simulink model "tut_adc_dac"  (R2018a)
settings: Solver=VariableStepAuto  StartTime=0.0  StopTime=10.0  RelTol=1e-3
undefined symbols (not defined in the file): adc_data_ch1, adc_data_ch2, adc_data_valid, Bit, Both, bram, c, d, hex2dec, led, Location, Lower, Minimum_Area, out, RED_PITAYA_10, reg, ROACH, ROACH2, rst_cntrl, Unsigned, Upper, Width, xc7z010
libraries: xbsIndex_r4 x149, xps_library x6, casper_library_misc x2
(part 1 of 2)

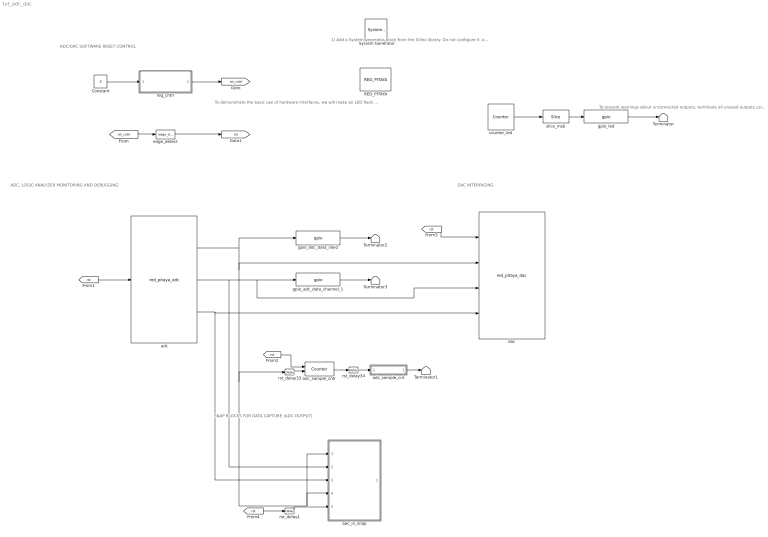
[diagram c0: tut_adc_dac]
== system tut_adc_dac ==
  note: 1) Add a System generator block from the Xilinx library. Do not configure it, add an "XSG core config" to do this for you. 2) Add XSG core config block from the CASPER XPS Blockset. Set it for SKARAB:xc7vx690t with sysclk. sys_clk is an onboard 156.25MHz crystal.
  note: To demonstrate the basic use of hardware interfaces, we will make an LED flash. With the FPGA running at a frequency > 156.25MHz, the most significant bit (msb) of a 27 bit counter will toggle approximately every 1.164 seconds (or quicker). Add a counter (Xilinx Blockset -> Basic Elements -> Counter). Set it for free running, 27 bits, unsigned. Add a slice block to select out the msb (Xilinx Blockset -> Basic Elements -> Slice). Set it for 1 bit wide with offset from top bit at zero. Add a GPIO block (CASPER XPS Blockset -> gpio). Set it to use the Red Pitaya LED bank as output, GPIO bit index 0 (the first LED).
  note: To prevent warnings about unconnected outputs, terminate all unused outputs using a Terminator: Simulink -> Sinks -> Terminator"
  note: ADC/DAC SOFTWARE RESET CONTROL
  note: ADC, LOGIC ANALYZER MONITORING AND DEBUGGING
  note: DAC INTERFACING
  note: SNAP BLOCKS FOR DATA CAPTURE (ADC OUTPUT)
  " System Generator" : xbsIndex_r4/ System Generator  Tag=genX  xilinxfamily=zynq  part=xc7z010  speed=-1  package=clg400  synthesis_tool=XST  clock_wrapper=Clock Enables  directory=/home/hpw1/work/tutorials_devel/vivado_2018/red_pitaya/tut_adc_dac/tut_adc_dac/sysgen  proj_type=Vivado  Synth_file=Vivado Synthesis Defaults  Impl_file=Vivado Implementation Defaults  testbench=off  simulink_period=1  sysclk_period=8  dcm_input_clock_period=10  incr_netlist=off  trim_vbits=Everywhere in SubSystem  dbl_ovrd=According to Block Masks  core_generation=According to Block Masks  run_coregen=off  deprecated_control=off  eval_field=0  block_type=sysgen
  Constant : Constant  Value=0
  RED_PITAYA : xps_library/Platforms/RED_PITAYA  Tag=xps:xsg  hw_sys=RED_PITAYA_10:xc7z010  clk_src=sys_clk  clk_rate=125  sample_period=1  synthesis_tool=XST
  Terminator{,1..3} (4 alike) : Terminator
  adc : xps_library/ADCs/red_pitaya_adc  Tag=xps:red_pitaya_adc  bits=10
  adc_in_snap : Subsystem  Tag=casper:bitsnap  AncestorBlock=casper_library_scopes/bitfield_snapshot  mask(bitsnap){io_names=[adc_data_valid adc_data_ch1 adc_data_ch2], io_widths=[1 10 10], io_bps=0, io_types=[2 1 1], show_format=on, snap_storage=bram, snap_dram_dimm=2, snap_dram_clock=250, snap_nsamples=10, snap_data_width=32, snap_offset=off, snap_circap=off, snap_value=off, snap_ext_arm=off, snap_ext_circ=off, snap_provide_outputs=on, snap_use_dsp48=on, snap_delay=0, extra_names=[c d], extra_widths=[30 2], extra_bps=[0 0], extra_types=[0 0]}
      mask prompts: io_names "Names [msb...lsb]"; io_widths "Bitwidths [msb...lsb]"; io_bps "Binary pts [msb...lsb]"; io_types "Data types [msb...lsb], ufix=0, fix=1, bool=2"; show_format "Print format string?"; snap_storage "Storage medium"; snap_dram_dimm "DRAM dimm"; snap_dram_clock "DRAM clock rate"; snap_nsamples "Number of Samples (2^?)"; snap_data_width "Data width"; snap_offset "Start delay support"; snap_circap "Circular capture support"; snap_value "Extra value capture support"; snap_ext_arm "External arm support"; snap_ext_circ "External circular capture support"; snap_provide_outputs "Provide outputs"; snap_use_dsp48 "Use DSP48s to implement counters"; snap_delay "Pre-snapshot delay"; extra_names "Names [msb...lsb]"; extra_widths "Widths [msb...lsb]"; extra_bps "Binary pts [msb...lsb]"; extra_types "Data types [msb...lsb], ufix=0, fix=1, bool=2"
      mask help: A wrapped snapshot block. Allows specification of inputs to a snapblock word so the toolflow can automatically set up the scope. See documentation for snapshot for explanation of parameters.
      mask init:
      | bitsnap_init(gcb);
  adc_sample_cnt : Subsystem  Tag=xps:sw_reg  AncestorBlock=xps_library/Memory/software_register  mask(swreg){io_dir=To Processor, io_delay=0, init_val=0, sample_period=1, names=reg, bitwidths=32, bin_pts=0, arith_types=0, sim_port=on, show_format=on}
      mask prompts: io_dir "I/O direction"; io_delay "I/O delay"; init_val "Initial Value"; sample_period "Sample period"; names "Bitfield names [msb...lsb]"; bitwidths "Bitfield widths"; bin_pts "Bitfield binary pts"; arith_types "Bitfield types, ufix=0, fix=1, bool=2"; sim_port "Provide sim input/output?"; show_format "Print format string?"
      mask help: A 32-bit software-accessible register. Can be divided into bitfields of varying widths and types using the fields in the block mask.
      mask init:
      | swreg_init(gcb)
  adc_sample_cntr : xbsIndex_r4/Counter  cnt_type=Free Running  cnt_to=1  operation=Up  start_count=0  cnt_by_val=1  arith_type=Unsigned  n_bits=32  bin_pt=0  load_pin=off  rst=on  en=on  explicit_period=on  period=1  use_behavioral_HDL=off  implementation=Fabric  use_rpm=off  dbl_ovrd=off  block_type=counter
  counter_led : xbsIndex_r4/Counter  cnt_type=Free Running  cnt_to=Inf  operation=Up  start_count=0  cnt_by_val=1  arith_type=Unsigned  n_bits=27  bin_pt=0  load_pin=off  rst=off  en=off  explicit_period=on  period=1  use_behavioral_HDL=off  implementation=Fabric  dbl_ovrd=off  block_type=counter
  dac : xps_library/DACs/red_pitaya_dac  Tag=xps:red_pitaya_dac  bits=10
  edge_detect : casper_library_misc/edge_detect  edge=Rising  polarity=Active High  x_in=[0 0.08 0.08 0.16 0.16 0.24 0.24 0.32 0.32 0.4]  y_in="[-1 -1  1  1  1  1  1  1  1  1]"  x_out=[0.6 0.68 0.68 0.76 0.76 0.84 0.84 0.92 0.92 1]  y_out="[-1 -1  1  1 -1 -1 -1 -1 -1 -1]"
  gpio_adc_data_channel_1 : xps_library/IO/gpio  Tag=xps:gpio  io_group_params_forwarded=off  io_group=ROACH:led  io_group_real=gpio  io_group_custom=0  io_dir=out  arith_type="Signed  (2's comp)"  bitwidth=10  bin_pt=0  bit_index=[0 1 2 3 4 5 6 7 8 9]  sample_period=1  use_single_ended=off  use_ddr=off  reg_iob=on  reg_clk_phase=0  termination=None
  gpio_adc_data_valid : xps_library/IO/gpio  Tag=xps:gpio  io_group_params_forwarded=off  io_group=ROACH:led  io_group_real=gpio  io_group_custom=0  io_dir=out  arith_type=Boolean  bitwidth=1  bin_pt=0  bit_index=10  sample_period=1  use_single_ended=off  use_ddr=off  reg_iob=on  reg_clk_phase=0  termination=None
  gpio_led : xps_library/IO/gpio  Tag=xps:gpio  io_group_params_forwarded=on  io_group=ROACH2:led  io_group_real=led  io_group_custom=0  io_dir=out  arith_type=Boolean  bitwidth=1  bin_pt=0  bit_index=0  sample_period=1  use_single_ended=off  use_ddr=off  reg_iob=on  reg_clk_phase=0  termination=None
  reg_cntrl : Subsystem  Tag=xps:sw_reg  AncestorBlock=xps_library/Memory/software_register  mask(swreg){io_dir=From Processor, io_delay=0, init_val=0, sample_period=1, names=rst_cntrl, bitwidths=[1], bin_pts=0, arith_types=[2], sim_port=on, show_format=on}
      mask prompts: io_dir "I/O direction"; io_delay "I/O delay"; init_val "Initial Value"; sample_period "Sample period"; names "Bitfield names [msb...lsb]"; bitwidths "Bitfield widths"; bin_pts "Bitfield binary pts"; arith_types "Bitfield types, ufix=0, fix=1, bool=2"; sim_port "Provide sim input/output?"; show_format "Print format string?"
      mask help: A 32-bit software-accessible register. Can be divided into bitfields of varying widths and types using the fields in the block mask.
      mask init:
      | swreg_init(gcb)
  rst_delay1 : xbsIndex_r4/Delay  rst=off  infoeditControl=Selection of Reset will increase slice count due to use of real FFs and instead of SRLs  en=off  latency=1  reg_retiming=on  dbl_ovrd=off  block_type=delay
  rst_delay33 : xbsIndex_r4/Delay  rst=off  infoeditControl=Selection of Reset will increase slice count due to use of real FFs and instead of SRLs  en=off  latency=2  reg_retiming=on  dbl_ovrd=off  block_type=delay
  rst_delay34 : xbsIndex_r4/Delay  rst=off  infoeditControl=Selection of Reset will increase slice count due to use of real FFs and instead of SRLs  en=off  latency=2  reg_retiming=on  dbl_ovrd=off  block_type=delay
  slice_msb : xbsIndex_r4/Slice  nbits=1  boolean_output=off  mode=Upper Bit Location + Width  bit1=0  base1=MSB of Input  bit0=0  base0=LSB of Input  dbl_ovrd=off  block_type=slice
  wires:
  gpio_led/1 -> Terminator/1
  counter_led/1 -> slice_msb/1
  slice_msb/1 -> gpio_led/1
  Constant/1 -> reg_cntrl/1(sim_1)
  reg_cntrl/1(in_rst_cntrl) -> [rst_cntrl]
  [rst_cntrl] -> edge_detect/1
  edge_detect/1 -> [rst]
  [rst] -> adc/1
  rst_delay34/1 -> adc_sample_cnt/1(out_reg)
  rst_delay33/1 -> adc_sample_cntr/2
  adc_sample_cnt/1(sim_out) -> Terminator1/1
  adc_sample_cntr/1 -> rst_delay34/1
  [rst] -> adc_sample_cntr/1
  adc/1 -> gpio_adc_data_valid/1, adc_in_snap/1(in_adc_data_valid), adc_in_snap/4(we), rst_delay33/1, dac/2
  gpio_adc_data_valid/1 -> Terminator2/1
  gpio_adc_data_channel_1/1 -> Terminator3/1
  [rst] -> dac/1
  rst_delay1/1 -> adc_in_snap/5(trig)
  [rst] -> rst_delay1/1
  adc/2 -> adc_in_snap/2(in_adc_data_ch1), dac/3, gpio_adc_data_channel_1/1
  adc/3 -> adc_in_snap/3(in_adc_data_ch2), dac/4

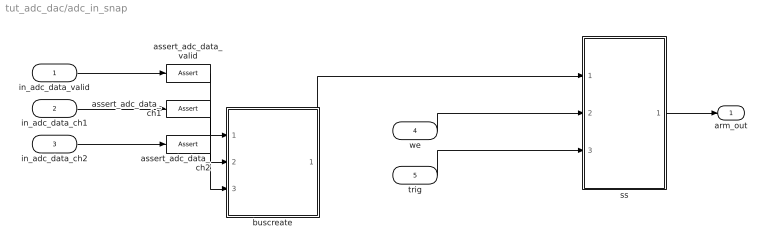
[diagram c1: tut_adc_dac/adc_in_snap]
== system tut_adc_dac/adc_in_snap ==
  in_adc_data_valid : Inport
  in_adc_data_ch1 : Inport  Port=2
  in_adc_data_ch2 : Inport  Port=3
  we : Inport  Port=4
  trig : Inport  Port=5
  assert_adc_data_ch1 : xbsIndex_r4/Assert  assert_type=on  type_source=Explicitly  gui_display_data_type=Fixed-point  arith_type="Signed  (2's comp)"  n_bits=10  bin_pt=0  preci_type=Single  exp_width=8  frac_width=24  assert_rate=off  rate_source=Explicitly  period=1  output_port=on  block_type=assert
  assert_adc_data_ch2 : xbsIndex_r4/Assert  assert_type=on  type_source=Explicitly  gui_display_data_type=Fixed-point  arith_type="Signed  (2's comp)"  n_bits=10  bin_pt=0  preci_type=Single  exp_width=8  frac_width=24  assert_rate=off  rate_source=Explicitly  period=1  output_port=on  block_type=assert
  assert_adc_data_valid : xbsIndex_r4/Assert  assert_type=on  type_source=Explicitly  gui_display_data_type=Boolean  arith_type=Boolean  n_bits=1  bin_pt=0  preci_type=Single  exp_width=8  frac_width=24  assert_rate=off  rate_source=Explicitly  period=1  output_port=on  block_type=assert
  buscreate : Subsystem  AncestorBlock=casper_library_flow_control/bus_create  mask(bus_create){inputNum=3}
      mask prompts: inputNum "Number of inputs:"
      mask init:
      | bus_create_init(gcb,...
      |     'inputNum', inputNum);
  ss : Subsystem  Tag=casper:snapshot  AncestorBlock=casper_library_scopes/snapshot  mask(snapshot){storage=bram, dram_dimm=2, dram_clock=250, nsamples=10, data_width=32, offset=off, circap=off, value=off, ext_arm=off, ext_circ=off, provide_outputs=off, use_dsp48=on}
      mask prompts: storage "Storage medium"; dram_dimm "DRAM dimm"; dram_clock "DRAM clock rate"; nsamples "Number of Samples (2^?)"; data_width "Data width"; offset "Start delay support"; circap "Circular capture support"; value "Extra value capture support"; ext_arm "External arm support"; ext_circ "External circular capture support"; provide_outputs "Provide outputs"; use_dsp48 "Use DSP48s to implement counters"
      mask help: Standard snap block, but with the following optional extras; 1) Optionally delay the fabric trigger by a user-specified number of valids. 2) Capture continuously after a trigger until a stop pulse is received. Data is captured into BRAM continuously, with old data being overwritten until a stop command is received. Then stop capturing when memory is filled. This enables you to get some data before and some data after the stop pulse. Use the 'tr_en_cnt' register to determine where you are in your vector. 'Addr' register's MSb now indicates 'busy capturing'. 3) Optionally capture a value on an i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
      mask init:
      | snapshot_init(gcb, ...
      |     'storage', storage, ...
      |     'dram_dimm', dram_dimm, ...
      |     'dram_clock', dram_clock, ...
      |     'nsamples', nsamples, ...
      |     'data_width', data_width, ...
      |     'offset', offset, ...
      |     'circap', circap, ...
      |     'value', value, ...
      |     'ext_arm', ext_arm, ...
      |     'ext_circ', ext_circ, ...
      |     'provide_outputs', 'off', ...
      |     'use_dsp48', use_dsp48);
  arm_out : Outport
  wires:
  ss/1(arm_out) -> arm_out/1
  buscreate/1(bus_out) -> ss/1(din)
  in_adc_data_valid/1 -> assert_adc_data_valid/1
  assert_adc_data_valid/1 -> buscreate/1(in1)
  in_adc_data_ch1/1 -> assert_adc_data_ch1/1
  assert_adc_data_ch1/1 -> buscreate/2(in2)
  in_adc_data_ch2/1 -> assert_adc_data_ch2/1
  assert_adc_data_ch2/1 -> buscreate/3(in3)
  we/1 -> ss/2(we)
  trig/1 -> ss/3(trig)

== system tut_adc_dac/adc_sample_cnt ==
  out_reg : Inport
  assert_reg : xbsIndex_r4/Assert  assert_type=on  type_source=Explicitly  gui_display_data_type=Fixed-point  arith_type=Unsigned  n_bits=32  bin_pt=0  preci_type=Single  exp_width=8  frac_width=24  assert_rate=off  rate_source=Explicitly  period=1  output_port=on  block_type=assert
  cast_gw : xbsIndex_r4/Convert  gui_display_data_type=Fixed-point  arith_type=Unsigned  n_bits=32  bin_pt=0  float_type=Single  exp_bits=8  fraction_bits=24  quantization=Truncate  overflow=Wrap  en=off  latency=1  pipeline=off  dbl_ovrd=off  block_type=convert
  io_delay : xbsIndex_r4/Delay  rst=off  infoeditControl=Selection of Reset will increase slice count due to use of real FFs and instead of SRLs  en=off  latency=0  reg_retiming=on  dbl_ovrd=off  block_type=delay
  reint1 : xbsIndex_r4/Reinterpret  force_arith_type=on  arith_type=Unsigned  force_bin_pt=on  bin_pt=0  block_type=reinterpret
  tut_adc_dac_adc_sample_cnt_user_data_in : xbsIndex_r4/Gateway Out  inherit_from_input=off  hdl_port=on  rows=1  columns=1  UseAsDAC=off  DACChannel='1'  interface=None  automatic_assignment=on  address_offset=hex2dec('00')  intf_name=''  intf_description=''  timing_constraint=None  locs_specified=off  LOCs={}  io_standard={}  block_type=gatewayout
  sim_out : Outport
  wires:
  io_delay/1 -> cast_gw/1
  cast_gw/1 -> tut_adc_dac_adc_sample_cnt_user_data_in/1
  tut_adc_dac_adc_sample_cnt_user_data_in/1 -> sim_out/1
  out_reg/1 -> assert_reg/1
  assert_reg/1 -> reint1/1
  reint1/1 -> io_delay/1

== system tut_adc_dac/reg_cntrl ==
  sim_1 : Inport
  convert1_1 : DataTypeConversion  OutDataTypeStr=fixdt('ufix1_En0')
  convert2_1 : DataTypeConversion  OutDataTypeStr=fixdt('ufix1_En0')  ConvertRealWorld=Stored Integer (SI)
  gain_1 : Gain
  io_delay : xbsIndex_r4/Delay  rst=off  infoeditControl=Selection of Reset will increase slice count due to use of real FFs and instead of SRLs  en=off  latency=0  reg_retiming=on  dbl_ovrd=off  block_type=delay
  slice_rst_cntrl : xbsIndex_r4/Slice  nbits=1  boolean_output=on  mode=Lower Bit Location + Width  bit1=0  base1=MSB of Input  bit0=0  base0=LSB of Input  dbl_ovrd=off  block_type=slice
  tut_adc_dac_reg_cntrl_user_data_out : xbsIndex_r4/Gateway In  gui_display_data_type=Fixed-point  arith_type=Unsigned  n_bits=32  bin_pt=0  preci_type=Single  exp_width=8  frac_width=24  rows=1  columns=1  quantization="Round  (unbiased: +/- Inf)"  overflow=Saturate  period=1  UseAsADC=off  ADCChannel='1'  interface=None  automatic_assignment=on  address_offset=hex2dec('00')  intf_name=''  intf_description=''  default_value=0  timing_constraint=None  locs_specified=off  LOCs={}  io_standard={}  inherit_from_input=off  hdl_port=on  dbl_ovrd=off  block_type=gatewayin
  in_rst_cntrl : Outport
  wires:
  tut_adc_dac_reg_cntrl_user_data_out/1 -> io_delay/1
  sim_1/1 -> convert1_1/1
  convert1_1/1 -> convert2_1/1
  convert2_1/1 -> gain_1/1
  gain_1/1 -> tut_adc_dac_reg_cntrl_user_data_out/1
  io_delay/1 -> slice_rst_cntrl/1
  slice_rst_cntrl/1 -> in_rst_cntrl/1

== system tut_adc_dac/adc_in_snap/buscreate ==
  in1 : Inport
  in2 : Inport  Port=2
  in3 : Inport  Port=3
  concatenate : xbsIndex_r4/Concat  num_inputs=3  dbl_ovrd=off  block_type=concat
  reinterpret1 : xbsIndex_r4/Reinterpret  force_arith_type=on  arith_type=Unsigned  force_bin_pt=on  bin_pt=0  block_type=reinterpret
  reinterpret2 : xbsIndex_r4/Reinterpret  force_arith_type=on  arith_type=Unsigned  force_bin_pt=on  bin_pt=0  block_type=reinterpret
  reinterpret3 : xbsIndex_r4/Reinterpret  force_arith_type=on  arith_type=Unsigned  force_bin_pt=on  bin_pt=0  block_type=reinterpret
  bus_out : Outport
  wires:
  concatenate/1 -> bus_out/1
  in1/1 -> reinterpret1/1
  reinterpret1/1 -> concatenate/1
  in2/1 -> reinterpret2/1
  reinterpret2/1 -> concatenate/2
  in3/1 -> reinterpret3/1
  reinterpret3/1 -> concatenate/3

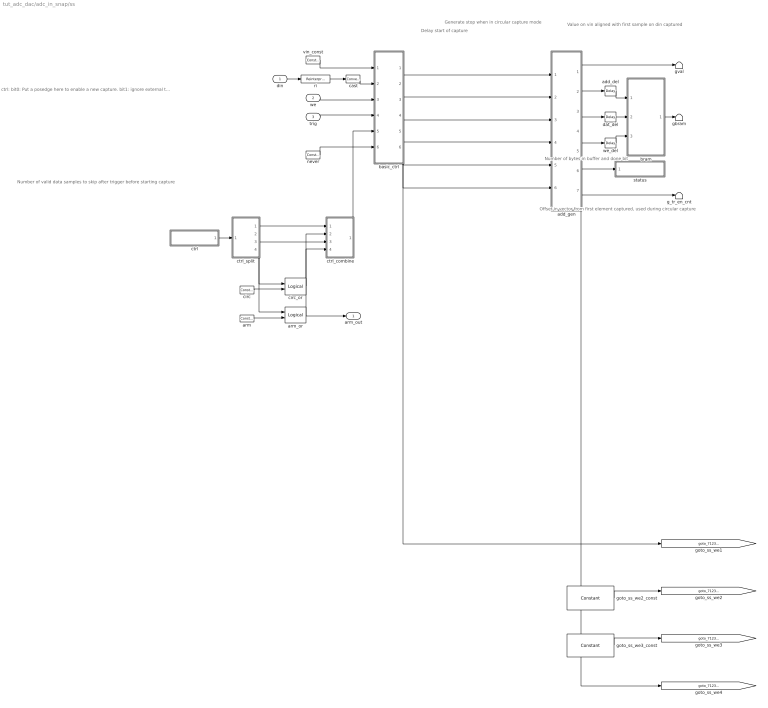
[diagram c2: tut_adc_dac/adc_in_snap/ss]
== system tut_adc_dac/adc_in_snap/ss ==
  note: Generate stop when in circular capture mode
  note: Delay start of capture
  note: ctrl: bit0: Put a posedge here to enable a new capture. bit1: ignore external trigger and trigger immediately. bit2: ignore external write enable and capture on every FPGA clock. bit3: continuously capture data until we get an external stop command.
  note: Offset in vector from first element captured, used during circular capture
  note: Number of bytes in buffer and done bit
  note: Number of valid data samples to skip after trigger before starting capture
  note: Value on vin aligned with first sample on din captured
  din : Inport
  we : Inport  Port=2
  trig : Inport  Port=3
  add_del : xbsIndex_r4/Delay  rst=off  infoeditControl=Selection of Reset will increase slice count due to use of real FFs and instead of SRLs  en=off  latency=1  reg_retiming=on  dbl_ovrd=off  block_type=delay
  add_gen : Subsystem  AncestorBlock=casper_library_scopes/snapshot/add_gen  mask{counter_size=10+2+1, increment=4, nsamples=10, burst_size=0, use_dsp48=on}
      mask prompts: counter_size "Address counter size (2^?)"; increment "Address counter increment"; nsamples "Number of samples (2^?)"; burst_size "Burst size (2^?)"; use_dsp48 "dsp48 counter/s"
      mask init:
      | set_param(gcb,'LinkStatus','inactive');
      | if strcmp(use_dsp48,'on'),
      |     set_param([gcb,'/add_gen'],'implementation','DSP48');
      | else
      |     set_param([gcb,'/add_gen'],'implementation','Fabric');
      | end
  arm : xbsIndex_r4/Constant  const=0  gui_display_data_type=Fixed-point  arith_type=Boolean  n_bits=16  bin_pt=14  preci_type=Single  exp_width=8  frac_width=24  explicit_period=on  period=1  equ=P=C  opselect=C  inp2=PCIN>>17  opr=+  inp1=P  carry=CIN  dbl_ovrd=off  block_type=constant
  arm_or : xbsIndex_r4/Logical  logical_function=OR  inputs=2  en=off  latency=0  precision=Full  arith_type=Unsigned  n_bits=16  bin_pt=0  align_bp=on  dbl_ovrd=off  block_type=logical
  basic_ctrl : Subsystem  AncestorBlock=casper_library_scopes/snapshot/basic_ctrl  mask{dram=off, data_width=32}
      mask prompts: data_width "data width"
      mask init:
      | set_param(gcb,'LinkStatus','inactive');
      | set_param([gcb,'/dram_munge'], 'dram', dram);
  bram : Subsystem  Tag=xps:bram  AncestorBlock=xps_library/Memory/shared_bram  mask{arith_type=Unsigned, addr_width=10, data_width=32, reg_prim_output=off, reg_core_output=off, optimization=Minimum_Area, data_bin_pt=0, init_vals=[0:2^10-1], sample_rate=1}
      mask prompts: arith_type "Output Data Type"; addr_width "Address width"; data_width "Data Width"; reg_prim_output "Register Primitive Output"; reg_core_output "Register Core Output"; data_bin_pt "Data Binary Point"; init_vals "Initial values (simulation only)"; sample_rate "Sample rate"
      mask init:
      | shared_bram_mask;
  cast : xbsIndex_r4/Convert  gui_display_data_type=Fixed-point  arith_type=Unsigned  n_bits=32  bin_pt=0  float_type=Single  exp_bits=8  fraction_bits=24  quantization=Truncate  overflow=Wrap  en=off  latency=0  pipeline=off  dbl_ovrd=off  block_type=convert
  circ : xbsIndex_r4/Constant  const=0  gui_display_data_type=Fixed-point  arith_type=Boolean  n_bits=16  bin_pt=14  preci_type=Single  exp_width=8  frac_width=24  explicit_period=on  period=1  equ=P=C  opselect=C  inp2=PCIN>>17  opr=+  inp1=P  carry=CIN  dbl_ovrd=off  block_type=constant
  circ_or : xbsIndex_r4/Logical  logical_function=OR  inputs=2  en=off  latency=0  precision=Full  arith_type=Unsigned  n_bits=16  bin_pt=0  align_bp=on  dbl_ovrd=off  block_type=logical
  ctrl : Subsystem  Tag=xps:sw_reg  AncestorBlock=xps_library/Memory/software_register  mask(swreg){io_dir=From Processor, io_delay=0, init_val=0, sample_period=1, names=reg, bitwidths=32, bin_pts=0, arith_types=0, sim_port=off, show_format=on}
      mask prompts: io_dir "I/O direction"; io_delay "I/O delay"; init_val "Initial Value"; sample_period "Sample period"; names "Bitfield names [msb...lsb]"; bitwidths "Bitfield widths"; bin_pts "Bitfield binary pts"; arith_types "Bitfield types, ufix=0, fix=1, bool=2"; sim_port "Provide sim input/output?"; show_format "Print format string?"
      mask help: A 32-bit software-accessible register. Can be divided into bitfields of varying widths and types using the fields in the block mask.
      mask init:
      | swreg_init(gcb)
  ctrl_combine : Subsystem  AncestorBlock=casper_library_flow_control/bus_create  mask(bus_create){inputNum=4}
      mask prompts: inputNum "Number of inputs:"
      mask init:
      | bus_create_init(gcb,...
      |     'inputNum', inputNum);
  ctrl_split : Subsystem  AncestorBlock=casper_library_flow_control/bus_expand  mask(bus_expand){mode=divisions of arbitrary size, outputNum=1, outputWidth=[28 1 2 1], outputBinaryPt=0, outputArithmeticType=[0 2 0 2], show_format=on, outputToWorkspace=off, variablePrefix=out, outputToModelAsWell=on}
      mask prompts: outputNum "Number of outputs:"; outputWidth "Output width [msb ... lsb]:"; outputBinaryPt "Output binary point position [msb ... lsb]:"; outputArithmeticType "Output arithmetic type (ufix=0, fix=1, bool=2) [msb ... lsb]:"; show_format "Print format string?"; outputToWorkspace "Output to workspace?"; variablePrefix "Variable name prefix:"; outputToModelAsWell "Output to model as well?"
      mask help: Expands a 'bus' made using a bus_create or Xilinx concat block. The input will be divided into the specified number of outputs with the specified arithmetic types. Divisions are made from most significant bit.
      mask init:
      | bus_expand_init(gcb,...
      |     'mode', mode, ...
      |     'outputNum', outputNum, ...
      |     'outputWidth', outputWidth, ...
      |     'outputBinaryPt', outputBinaryPt, ...
      |     'outputArithmeticType', outputArithmeticType, ...
      |     'show_format', show_format, ...
      |     'outputToWorkspace', outputToWorkspace, ...
      |     'variablePrefix', variablePrefix, ...
      |     'outputToModelAsWell', outputToModelAsWell);
  dat_del : xbsIndex_r4/Delay  rst=off  infoeditControl=Selection of Reset will increase slice count due to use of real FFs and instead of SRLs  en=off  latency=1  reg_retiming=on  dbl_ovrd=off  block_type=delay
  g_tr_en_cnt : Terminator
  gbram : Terminator
  goto_ss_we2_const : xbsIndex_r4/Constant  const=0  gui_display_data_type=Fixed-point  arith_type=Boolean  n_bits=16  bin_pt=14  preci_type=Single  exp_width=8  frac_width=24  explicit_period=on  period=1  equ=P=C  opselect=C  inp2=PCIN>>17  opr=+  inp1=P  carry=CIN  dbl_ovrd=off  block_type=constant
  goto_ss_we3_const : xbsIndex_r4/Constant  const=0  gui_display_data_type=Fixed-point  arith_type=Boolean  n_bits=16  bin_pt=14  preci_type=Single  exp_width=8  frac_width=24  explicit_period=on  period=1  equ=P=C  opselect=C  inp2=PCIN>>17  opr=+  inp1=P  carry=CIN  dbl_ovrd=off  block_type=constant
  gval : Terminator
  never : xbsIndex_r4/Constant  const=0  gui_display_data_type=Fixed-point  arith_type=Boolean  n_bits=16  bin_pt=14  preci_type=Single  exp_width=8  frac_width=24  explicit_period=on  period=1  equ=P=C  opselect=C  inp2=PCIN>>17  opr=+  inp1=P  carry=CIN  dbl_ovrd=off  block_type=constant
  ri : xbsIndex_r4/Reinterpret  force_arith_type=on  arith_type=Unsigned  force_bin_pt=on  bin_pt=0  block_type=reinterpret
  status : Subsystem  Tag=xps:sw_reg  AncestorBlock=xps_library/Memory/software_register  mask(swreg){io_dir=To Processor, io_delay=0, init_val=0, sample_period=1, names=reg, bitwidths=32, bin_pts=0, arith_types=0, sim_port=off, show_format=on}
      mask prompts: io_dir "I/O direction"; io_delay "I/O delay"; init_val "Initial Value"; sample_period "Sample period"; names "Bitfield names [msb...lsb]"; bitwidths "Bitfield widths"; bin_pts "Bitfield binary pts"; arith_types "Bitfield types, ufix=0, fix=1, bool=2"; sim_port "Provide sim input/output?"; show_format "Print format string?"
      mask help: A 32-bit software-accessible register. Can be divided into bitfields of varying widths and types using the fields in the block mask.
      mask init:
      | swreg_init(gcb)
  vin_const : xbsIndex_r4/Constant  const=0  gui_display_data_type=Fixed-point  arith_type=Boolean  n_bits=16  bin_pt=14  preci_type=Single  exp_width=8  frac_width=24  explicit_period=on  period=1  equ=P=C  opselect=C  inp2=PCIN>>17  opr=+  inp1=P  carry=CIN  dbl_ovrd=off  block_type=constant
  we_del : xbsIndex_r4/Delay  rst=off  infoeditControl=Selection of Reset will increase slice count due to use of real FFs and instead of SRLs  en=off  latency=1  reg_retiming=on  dbl_ovrd=off  block_type=delay
  arm_out : Outport
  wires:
  din/1 -> ri/1
  ri/1 -> cast/1
  cast/1 -> basic_ctrl/2(din)
  we/1 -> basic_ctrl/3(we)
  trig/1 -> basic_ctrl/4(trig)
  ctrl_combine/1(bus_out) -> basic_ctrl/5(ctrl)
  never/1 -> basic_ctrl/6(stopi)
  arm/1 -> arm_or/2
  arm_or/1 -> arm_out/1, ctrl_combine/4(in4)
  circ/1 -> circ_or/2
  ctrl/1(in_reg) -> ctrl_split/1(bus_in)
  ctrl_split/1(msb_out4) -> ctrl_combine/1(in1)
  ctrl_split/2(out3) -> circ_or/1
  ctrl_split/3(out2) -> ctrl_combine/3(in3)
  ctrl_split/4(lsb_out1) -> arm_or/1
  circ_or/1 -> ctrl_combine/2(in2)
  basic_ctrl/1(vout) -> add_gen/1(vin)
  basic_ctrl/2(dout) -> add_gen/2(din)
  basic_ctrl/3(we_o) -> add_gen/3(we), [goto_71237712_we1]
  basic_ctrl/4(go) -> add_gen/4(go)
  basic_ctrl/5(stop) -> add_gen/5(cont)
  basic_ctrl/6(init) -> add_gen/6(init)
  add_gen/5(status) -> status/1(out_reg)
  vin_const/1 -> basic_ctrl/1(vin)
  add_gen/1(vout) -> gval/1
  add_gen/6(en_cnt) -> g_tr_en_cnt/1
  add_gen/2(add) -> add_del/1
  add_gen/3(dout) -> dat_del/1
  add_gen/4(we_o) -> we_del/1, [goto_71237712_we4]
  add_del/1 -> bram/1(addr)
  dat_del/1 -> bram/2(data_in)
  we_del/1 -> bram/3(we)
  bram/1(data_out) -> gbram/1
  goto_ss_we2_const/1 -> [goto_71237712_we2]
  goto_ss_we3_const/1 -> [goto_71237712_we3]

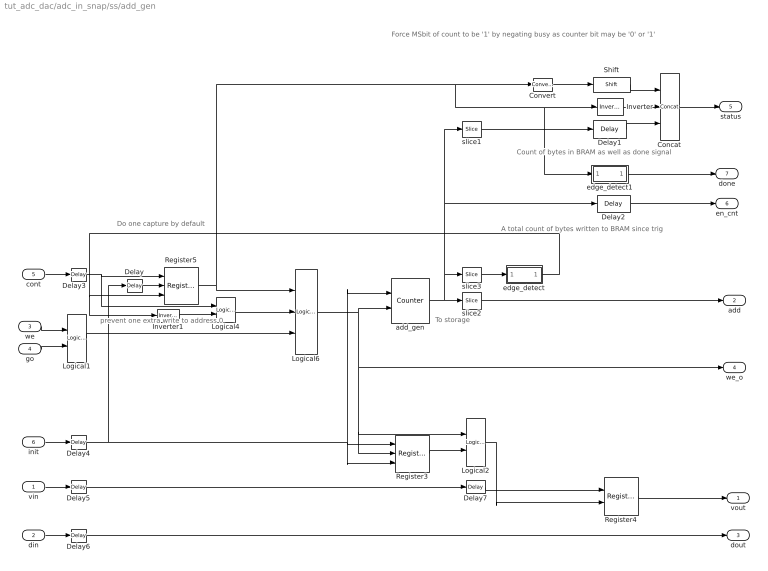
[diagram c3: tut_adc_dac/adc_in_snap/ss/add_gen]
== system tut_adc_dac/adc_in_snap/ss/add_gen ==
  note: Force MSbit of count to be '1' by negating busy as counter bit may be '0' or '1'
  note: A total count of bytes written to BRAM since trig
  note: Count of bytes in BRAM as well as done signal
  note: Do one capture by default
  note: prevent one extra write to address 0
  note: To storage
  vin : Inport
  din : Inport  Port=2
  we : Inport  Port=3
  go : Inport  Port=4
  cont : Inport  Port=5
  init : Inport  Port=6
  Concat : xbsIndex_r4/Concat  num_inputs=3  dbl_ovrd=off  block_type=concat
  Convert : xbsIndex_r4/Convert  gui_display_data_type=Fixed-point  arith_type=Unsigned  n_bits=32-nsamples-log2(increment)-1  bin_pt=0  float_type=Single  exp_bits=8  fraction_bits=24  quantization=Truncate  overflow=Wrap  en=off  latency=0  pipeline=off  dbl_ovrd=off  block_type=convert
  Delay{,3..6} (5 alike) : xbsIndex_r4/Delay  rst=off  infoeditControl=Selection of Reset will increase slice count due to use of real FFs and instead of SRLs  en=off  latency=1  reg_retiming=on  dbl_ovrd=off  block_type=delay
  Delay1 : xbsIndex_r4/Delay  rst=off  infoeditControl=Selection of Reset will increase slice count due to use of real FFs and instead of SRLs  en=off  latency=1  reg_retiming=off  dbl_ovrd=off  block_type=delay
  Delay2 : xbsIndex_r4/Delay  rst=off  infoeditControl=Selection of Reset will increase slice count due to use of real FFs and instead of SRLs  en=off  latency=1  reg_retiming=off  dbl_ovrd=off  block_type=delay
  Delay7 : xbsIndex_r4/Delay  rst=off  infoeditControl=Selection of Reset will increase slice count due to use of real FFs and instead of SRLs  en=off  latency=1  reg_retiming=off  dbl_ovrd=off  block_type=delay
  Inverter : xbsIndex_r4/Inverter  en=off  latency=1  dbl_ovrd=off  block_type=inv
  Inverter1 : xbsIndex_r4/Inverter  en=off  latency=0  dbl_ovrd=off  block_type=inv
  Logical1 : xbsIndex_r4/Logical  logical_function=AND  inputs=2  en=off  latency=1  precision=Full  arith_type=Unsigned  n_bits=8  bin_pt=2  align_bp=on  dbl_ovrd=off  block_type=logical
  Logical2 : xbsIndex_r4/Logical  logical_function=AND  inputs=2  en=off  latency=1  precision=Full  arith_type=Unsigned  n_bits=8  bin_pt=2  align_bp=on  dbl_ovrd=off  block_type=logical
  Logical4 : xbsIndex_r4/Logical  logical_function=OR  inputs=2  en=off  latency=0  precision=Full  arith_type=Unsigned  n_bits=8  bin_pt=2  align_bp=on  dbl_ovrd=off  block_type=logical
  Logical6 : xbsIndex_r4/Logical  logical_function=AND  inputs=3  en=off  latency=0  precision=Full  arith_type=Unsigned  n_bits=8  bin_pt=2  align_bp=on  dbl_ovrd=off  block_type=logical
  Register3 : xbsIndex_r4/Register  init=0  rst=on  en=on  dbl_ovrd=off  block_type=register
  Register4 : xbsIndex_r4/Register  init=0  rst=off  en=on  dbl_ovrd=off  block_type=register
  Register5 : xbsIndex_r4/Register  init=1  rst=on  en=on  dbl_ovrd=off  block_type=register
  Shift : xbsIndex_r4/Shift  shift_dir=Left  shift_bits=32-nsamples-log2(increment)-1-1  en=off  latency=1  precision=Full  arith_type="Signed  (2's comp)"  n_bits=16  bin_pt=14  quantization=Truncate  overflow=Wrap  dbl_ovrd=off  block_type=shift
  add_gen : xbsIndex_r4/Counter  cnt_type=Free Running  cnt_to=1  operation=Up  start_count=0  cnt_by_val=increment  arith_type=Unsigned  n_bits=counter_size  bin_pt=0  load_pin=off  rst=on  en=on  explicit_period=on  period=1  use_behavioral_HDL=off  implementation=DSP48  use_rpm=on  dbl_ovrd=off  block_type=counter
  edge_detect : Subsystem  AncestorBlock=casper_library_misc/edge_detect  mask(edge_detect){edge=Both, polarity=Active High, x_in=[0 0.08 0.08 0.16 0.16 0.24 0.24 0.32 0.32 0.4], y_in=[-1 -1  1  1  1  1 -1 -1 -1 -1], x_out=[0.6 0.68 0.68 0.76 0.76 0.84 0.84 0.92 0.92 1], y_out=[-1 -1  1  1 -1 -1  1  1 -1 -1]}
      mask prompts: edge "Edge Type"; polarity "Output Polarity"; x_in "Input X Positions"; y_in "Input Y Positions"; x_out "Output X Positions"; y_out "Output Y Positions"
      mask help: Output is active for one-cycle after each edge of the specified type (i.e. rising, falling or both).
      mask init:
      | edge_detect_init(gcb,...
      |     'edge',edge,...
      |     'polarity',polarity,...
      |     'x_in',x_in,...
      |     'x_out',x_out,...
      |     'y_in',y_in,...
      |     'y_out',y_out);
      | 
      | x_in_num=str2num(getfield(getfield(get_param(gcb,'UserData'),'parameters'),'x_in'));
      | x_out_num=str2num(getfield(getfield(get_param(gcb,'UserData'),'parameters'),'x_out'));
      | y_in_num=str2num(getfield(getfield(get_param(gcb,'UserData'),'parameters'),'y_in'));
      | y_out_num=str2num(getfield(getfield(get_param(gcb,'UserData'),'parameters'),'y_out'));
  edge_detect1 : Subsystem  AncestorBlock=casper_library_scopes/snapshot/add_gen/edge_detect  mask(edge_detect){edge=Both, polarity=Active High, x_in=[0 0.08 0.08 0.16 0.16 0.24 0.24 0.32 0.32 0.4], y_in=[-1 -1  1  1  1  1 -1 -1 -1 -1], x_out=[0.6 0.68 0.68 0.76 0.76 0.84 0.84 0.92 0.92 1], y_out=[-1 -1  1  1 -1 -1  1  1 -1 -1]}
      mask prompts: edge "Edge Type"; polarity "Output Polarity"; x_in "Input X Positions"; y_in "Input Y Positions"; x_out "Output X Positions"; y_out "Output Y Positions"
      mask help: Output is active for one-cycle after each edge of the specified type (i.e. rising, falling or both).
      mask init:
      | edge_detect_init(gcb,...
      |     'edge',edge,...
      |     'polarity',polarity,...
      |     'x_in',x_in,...
      |     'x_out',x_out,...
      |     'y_in',y_in,...
      |     'y_out',y_out);
      | 
      | x_in_num=str2num(getfield(getfield(get_param(gcb,'UserData'),'parameters'),'x_in'));
      | x_out_num=str2num(getfield(getfield(get_param(gcb,'UserData'),'parameters'),'x_out'));
      | y_in_num=str2num(getfield(getfield(get_param(gcb,'UserData'),'parameters'),'y_in'));
      | y_out_num=str2num(getfield(getfield(get_param(gcb,'UserData'),'parameters'),'y_out'));
  slice1 : xbsIndex_r4/Slice  nbits=nsamples+log2(increment)  boolean_output=off  mode=Lower Bit Location + Width  bit1=0  base1=LSB of Input  bit0=0  base0=LSB of Input  dbl_ovrd=off  block_type=slice
  slice2 : xbsIndex_r4/Slice  nbits=nsamples-burst_size  boolean_output=off  mode=Lower Bit Location + Width  bit1=0  base1=LSB of Input  bit0=log2(increment)+burst_size  base0=LSB of Input  dbl_ovrd=off  block_type=slice
  slice3 : xbsIndex_r4/Slice  nbits=1  boolean_output=on  mode=Lower Bit Location + Width  bit1=0  base1=MSB of Input  bit0=nsamples + log2(increment)  base0=LSB of Input  dbl_ovrd=off  block_type=slice
  vout : Outport
  add : Outport  Port=2
  dout : Outport  Port=3
  we_o : Outport  Port=4
  status : Outport  Port=5
  en_cnt : Outport  Port=6
  done : Outport  Port=7
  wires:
  Delay6/1 -> dout/1
  Delay5/1 -> Delay7/1
  Delay4/1 -> Delay/1, Register3/1, Register3/3, add_gen/1
  Delay3/1 -> Register5/1, Logical4/1
  Delay7/1 -> Register4/1
  Logical1/1 -> Logical6/3
  go/1 -> Logical1/2
  we/1 -> Logical1/1
  Logical4/1 -> Logical6/2
  Inverter/1 -> Concat/2
  slice1/1 -> Delay1/1
  Delay1/1 -> Concat/3
  din/1 -> Delay6/1
  Delay2/1 -> en_cnt/1
  slice2/1 -> add/1
  Convert/1 -> Shift/1
  Concat/1 -> status/1
  Logical6/1 -> add_gen/2, Register3/2, Logical2/1, we_o/1
  init/1 -> Delay4/1
  slice3/1 -> edge_detect/1(in)
  Register5/1 -> Logical6/1, edge_detect1/1(in), Inverter/1, Convert/1
  add_gen/1 -> slice3/1, Delay2/1, slice1/1, slice2/1
  vin/1 -> Delay5/1
  Register3/1 -> Logical2/2
  Logical2/1 -> Register4/2
  Register4/1 -> vout/1
  edge_detect/1(out) -> Register5/3, Inverter1/1
  cont/1 -> Delay3/1
  Inverter1/1 -> Logical4/2
  Delay/1 -> Register5/2
  Shift/1 -> Concat/1
  edge_detect1/1(out) -> done/1

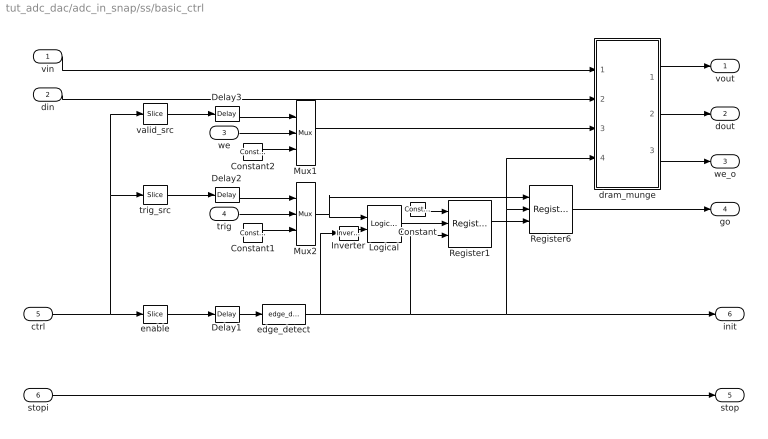
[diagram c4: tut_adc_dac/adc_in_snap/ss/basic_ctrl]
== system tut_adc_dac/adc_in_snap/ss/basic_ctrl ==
  vin : Inport
  din : Inport  Port=2
  we : Inport  Port=3
  trig : Inport  Port=4
  ctrl : Inport  Port=5
  stopi : Inport  Port=6
  Constant : xbsIndex_r4/Constant  const=1  gui_display_data_type=Fixed-point  arith_type=Boolean  n_bits=16  bin_pt=14  preci_type=Single  exp_width=8  frac_width=24  explicit_period=on  period=1  equ=P=C  opselect=C  inp2=PCIN>>17  opr=+  inp1=P  carry=CIN  dbl_ovrd=off  block_type=constant
  Constant1 : xbsIndex_r4/Constant  const=1  gui_display_data_type=Fixed-point  arith_type=Boolean  n_bits=1  bin_pt=0  preci_type=Single  exp_width=8  frac_width=24  explicit_period=on  period=1  equ=P=C  opselect=C  inp2=PCIN>>17  opr=+  inp1=P  carry=CIN  dbl_ovrd=off  block_type=constant
  Constant2 : xbsIndex_r4/Constant  const=1  gui_display_data_type=Fixed-point  arith_type=Boolean  n_bits=1  bin_pt=0  preci_type=Single  exp_width=8  frac_width=24  explicit_period=on  period=1  equ=P=C  opselect=C  inp2=PCIN>>17  opr=+  inp1=P  carry=CIN  dbl_ovrd=off  block_type=constant
  Delay1 : xbsIndex_r4/Delay  rst=off  infoeditControl=Selection of Reset will increase slice count due to use of real FFs and instead of SRLs  en=off  latency=1  reg_retiming=off  dbl_ovrd=off  block_type=delay
  Delay2 : xbsIndex_r4/Delay  rst=off  infoeditControl=Selection of Reset will increase slice count due to use of real FFs and instead of SRLs  en=off  latency=1  reg_retiming=off  dbl_ovrd=off  block_type=delay
  Delay3 : xbsIndex_r4/Delay  rst=off  infoeditControl=Selection of Reset will increase slice count due to use of real FFs and instead of SRLs  en=off  latency=1  reg_retiming=off  dbl_ovrd=off  block_type=delay
  Inverter : xbsIndex_r4/Inverter  en=off  latency=0  dbl_ovrd=off  block_type=inv
  Logical : xbsIndex_r4/Logical  logical_function=AND  inputs=2  en=off  latency=0  precision=Full  arith_type=Unsigned  n_bits=16  bin_pt=0  align_bp=on  dbl_ovrd=off  block_type=logical
  Mux1 : xbsIndex_r4/Mux  inputs=2  en=off  latency=0  precision=Full  arith_type="Signed  (2's comp)"  n_bits=8  bin_pt=2  quantization=Truncate  overflow=Wrap  dbl_ovrd=off  block_type=mux
  Mux2 : xbsIndex_r4/Mux  inputs=2  en=off  latency=0  precision=Full  arith_type="Signed  (2's comp)"  n_bits=8  bin_pt=2  quantization=Truncate  overflow=Wrap  dbl_ovrd=off  block_type=mux
  Register1 : xbsIndex_r4/Register  init=0  rst=on  en=on  dbl_ovrd=off  block_type=register
  Register6 : xbsIndex_r4/Register  init=0  rst=on  en=on  dbl_ovrd=off  block_type=register
  dram_munge : Subsystem  mask{dram=off, data_width=data_width}
      mask prompts: data_width "data width"
      mask init:
      | set_param(gcb,'LinkStatus','inactive');
      | if strcmp(dram,'on'),
      |     set_param([gcb,'/dram'], 'const', '1');
      | else,
      |     set_param([gcb,'/dram'], 'const', '0');
      | end
      | set_param([gcb,'/data_choice'], ...
      |         'precision', 'User Defined', ...
      |         'arith_type', 'Unsigned', ...
      |         'n_bits', num2str(data_width), 'bin_pt', '0', ...
      |         'quantization', 'Truncate', ...
      |         'overflow', 'Wrap');
  edge_detect : casper_library_misc/edge_detect  edge=Rising  polarity=Active High  x_in=[0 0.08 0.08 0.16 0.16 0.24 0.24 0.32 0.32 0.4]  y_in="[-1 -1  1  1  1  1  1  1  1  1]"  x_out=[0.6 0.68 0.68 0.76 0.76 0.84 0.84 0.92 0.92 1]  y_out="[-1 -1  1  1 -1 -1 -1 -1 -1 -1]"
      link override Delay: sg_icon_stat=45,16,1,1,white,blue,0,07b98262,right,,[ ],[ ]  sg_mask_display=fprintf('','COMMENT: begin icon graphics'); patch([0 45 45 0 0 ],[0 0 16 16 0 ],[0.77 0.82 0.91 ]); plot([0 45 45 0 0 ],[0 0 16 16 0 ]); patch([17.55 20.44 22.44 24.44 26.44 22.44 19.55 17.55 ],[10.22 10.22 12.22 10.22 12.22 12.22 12.22 10.22 ],[1 1 1 ]); patch([19.55 22.44 20.44 17.55 19.55 ],[8.22 8.22 10.22 10.22 8.22 ],[0.931 0.946 0.973 ]); patch([17.55 20.44 22.44 19.55 17.55 ],[6.22 6.22 8.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
      link override Inverter: sg_icon_stat=45,16,1,1,white,blue,0,267846e5,right,,[ ],[ ]  sg_mask_display=fprintf('','COMMENT: begin icon graphics'); patch([0 45 45 0 0 ],[0 0 16 16 0 ],[0.77 0.82 0.91 ]); plot([0 45 45 0 0 ],[0 0 16 16 0 ]); patch([17.55 20.44 22.44 24.44 26.44 22.44 19.55 17.55 ],[10.22 10.22 12.22 10.22 12.22 12.22 12.22 10.22 ],[1 1 1 ]); patch([19.55 22.44 20.44 17.55 19.55 ],[8.22 8.22 10.22 10.22 8.22 ],[0.931 0.946 0.973 ]); patch([17.55 20.44 22.44 19.55 17.55 ],[6.22 6.22 8.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
      link override edge_op: sg_icon_stat=45,44,2,1,white,blue,0,affe8783,right,,[ ],[ ]  sg_mask_display=fprintf('','COMMENT: begin icon graphics'); patch([0 45 45 0 0 ],[0 0 44 44 0 ],[0.77 0.82 0.91 ]); plot([0 45 45 0 0 ],[0 0 44 44 0 ]); patch([8.65 17.32 23.32 29.32 35.32 23.32 14.65 8.65 ],[28.66 28.66 34.66 28.66 34.66 34.66 34.66 28.66 ],[1 1 1 ]); patch([14.65 23.32 17.32 8.65 14.65 ],[22.66 22.66 28.66 28.66 22.66 ],[0.931 0.946 0.973 ]); patch([8.65 17.32 23.32 14.65 8.65 ],[16.66 16.66 22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
  enable : xbsIndex_r4/Slice  nbits=1  boolean_output=on  mode=Lower Bit Location + Width  bit1=0  base1=LSB of Input  bit0=0  base0=LSB of Input  dbl_ovrd=off  block_type=slice
  trig_src : xbsIndex_r4/Slice  nbits=1  boolean_output=on  mode=Lower Bit Location + Width  bit1=0  base1=LSB of Input  bit0=1  base0=LSB of Input  dbl_ovrd=off  block_type=slice
  valid_src : xbsIndex_r4/Slice  nbits=1  boolean_output=on  mode=Lower Bit Location + Width  bit1=0  base1=LSB of Input  bit0=2  base0=LSB of Input  dbl_ovrd=off  block_type=slice
  vout : Outport
  dout : Outport  Port=2
  we_o : Outport  Port=3
  go : Outport  Port=4
  stop : Outport  Port=5
  init : Outport  Port=6
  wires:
  Delay1/1 -> edge_detect/1
  Delay3/1 -> Mux1/1
  Delay2/1 -> Mux2/1
  dram_munge/1(vout) -> vout/1
  vin/1 -> dram_munge/1(vin)
  dram_munge/3(we_o) -> we_o/1
  dram_munge/2(dout) -> dout/1
  din/1 -> dram_munge/2(din)
  Inverter/1 -> Logical/2
  Mux2/1 -> Logical/1, Register6/1
  Register6/1 -> go/1
  trig/1 -> Mux2/2
  Mux1/1 -> dram_munge/3(we)
  we/1 -> Mux1/2
  ctrl/1 -> enable/1, valid_src/1, trig_src/1
  edge_detect/1 -> Inverter/1, Register1/3, dram_munge/4(init), Register6/2, init/1
  enable/1 -> Delay1/1
  Constant1/1 -> Mux2/3
  Constant2/1 -> Mux1/3
  trig_src/1 -> Delay2/1
  valid_src/1 -> Delay3/1
  Constant/1 -> Register1/1
  Register1/1 -> Register6/3
  Logical/1 -> Register1/2
  stopi/1 -> stop/1

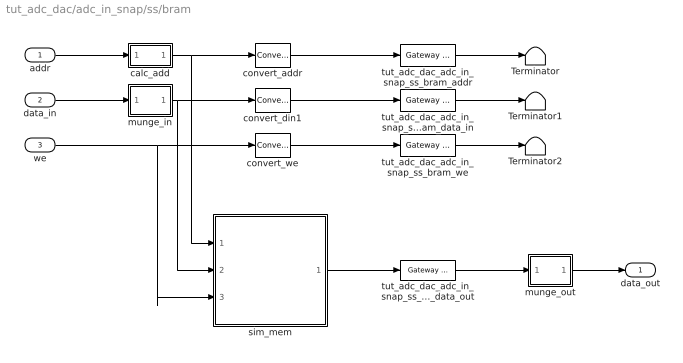
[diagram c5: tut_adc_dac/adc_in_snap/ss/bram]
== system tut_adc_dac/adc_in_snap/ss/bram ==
  addr : Inport
  data_in : Inport  Port=2
  we : Inport  Port=3
  Terminator : Terminator
  Terminator1 : Terminator
  Terminator2 : Terminator
  calc_add : Subsystem  mask{data_width=32, addr_width=10, sample_rate=sample_rate}
      mask prompts: data_width "data width"; addr_width "address width"; sample_rate "sample rate"
  convert_addr : xbsIndex_r4/Convert  gui_display_data_type=Fixed-point  arith_type=Unsigned  n_bits=addr_width  bin_pt=0  float_type=Single  exp_bits=8  fraction_bits=24  quantization=Truncate  overflow=Wrap  en=off  latency=0  pipeline=off  dbl_ovrd=off  block_type=convert
  convert_din1 : xbsIndex_r4/Convert  gui_display_data_type=Fixed-point  arith_type=Unsigned  n_bits=32  bin_pt=0  float_type=Single  exp_bits=8  fraction_bits=24  quantization=Truncate  overflow=Wrap  en=off  latency=0  pipeline=off  dbl_ovrd=off  block_type=convert
  convert_we : xbsIndex_r4/Convert  gui_display_data_type=Fixed-point  arith_type=Unsigned  n_bits=1  bin_pt=0  float_type=Single  exp_bits=8  fraction_bits=24  quantization=Truncate  overflow=Wrap  en=off  latency=0  pipeline=off  dbl_ovrd=off  block_type=convert
  munge_in : Subsystem  AncestorBlock=casper_library_flow_control/munge  mask(munge){divisions=1, div_size=32, order=[0], arith_type_out=Unsigned, bin_pt_out=0}
      mask prompts: divisions "Number of divisions"; div_size "Division size (bits)"; order "Division packing order"; arith_type_out "Output arithmetic type"; bin_pt_out "Output binary point"
      mask help: Splits an input bus into the specified number of divisions and then recombines them in the order specified (most significant division = 0,least = number divisions-1)
      mask init:
      | munge_init(gcb, ...
      |     'divisions', divisions, ...
      |     'div_size', div_size, ...
      |     'order', order, ...
      |     'arith_type_out', arith_type_out, ...
      |     'bin_pt_out', bin_pt_out);
  munge_out : Subsystem  AncestorBlock=casper_library_flow_control/munge  mask(munge){divisions=1, div_size=32, order=[0], arith_type_out=Unsigned, bin_pt_out=0}
      mask prompts: divisions "Number of divisions"; div_size "Division size (bits)"; order "Division packing order"; arith_type_out "Output arithmetic type"; bin_pt_out "Output binary point"
      mask help: Splits an input bus into the specified number of divisions and then recombines them in the order specified (most significant division = 0,least = number divisions-1)
      mask init:
      | munge_init(gcb, ...
      |     'divisions', divisions, ...
      |     'div_size', div_size, ...
      |     'order', order, ...
      |     'arith_type_out', arith_type_out, ...
      |     'bin_pt_out', bin_pt_out);
  sim_mem : Subsystem  mask{arith_type=Unsigned, addr_width=10, data_width=32, data_bin_pt=0, init_vals=[0     1     2     3     4     5     6     7     8     9    10    11    12    13    14    15    16    17    18    19    20    21    22    23    24    25    26    27    28    29    30    31    32    33    34    35    36    37    38    39    40    41    42    43    44    45    46    47    48    49    50    51    52    53    54    55    56    57    58    59    60    61    62    63    64    65    66  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, sample_rate=1, csp_latency=1}
      mask prompts: arith_type "Output Data Type"; addr_width "Address width"; data_width "Data width"; data_bin_pt "Data Binary Point"; init_vals "Initial values"; sample_rate "Sample rate"; csp_latency "Latency"
      mask init:
      | % set_param([gcb, '/data_to_xilinx'], 'arith_type', arith_type)
      | % set_param([gcb, '/data_to_xilinx'], 'n_bits', get_param(gcb, 'data_width'))
  tut_adc_dac_adc_in_snap_ss_bram_addr : xbsIndex_r4/Gateway Out  inherit_from_input=off  hdl_port=on  rows=1  columns=1  UseAsDAC=off  DACChannel='1'  interface=None  automatic_assignment=on  address_offset=hex2dec('00')  intf_name=''  intf_description=''  timing_constraint=None  locs_specified=off  LOCs={'A5','B9','A9','C1','A3','G6','E9','A6','A7','A8','B8','B1','B3','D9','B5','B4','B6','C2'}  io_standard={}  block_type=gatewayout
  tut_adc_dac_adc_in_snap_ss_bram_data_in : xbsIndex_r4/Gateway Out  inherit_from_input=off  hdl_port=on  rows=1  columns=1  UseAsDAC=off  DACChannel='1'  interface=None  automatic_assignment=on  address_offset=hex2dec('00')  intf_name=''  intf_description=''  timing_constraint=None  locs_specified=off  LOCs={'B21','B22','A22','B23','B19','C19','A20','A21','A23','B24','A24','A25','E18','D18','C18','B18'}  io_standard={}  block_type=gatewayout
  tut_adc_dac_adc_in_snap_ss_bram_data_out : xbsIndex_r4/Gateway In  gui_display_data_type=Fixed-point  arith_type=Unsigned  n_bits=32  bin_pt=0  preci_type=Single  exp_width=8  frac_width=24  rows=1  columns=1  quantization=Truncate  overflow=Wrap  period=sample_rate  UseAsADC=off  ADCChannel='1'  interface=None  automatic_assignment=on  address_offset=hex2dec('00')  intf_name=''  intf_description=''  default_value=0  timing_constraint=None  locs_specified=off  LOCs={}  io_standard={}  inherit_from_input=off  hdl_port=on  dbl_ovrd=off  block_type=gatewayin
  tut_adc_dac_adc_in_snap_ss_bram_we : xbsIndex_r4/Gateway Out  inherit_from_input=off  hdl_port=on  rows=1  columns=1  UseAsDAC=off  DACChannel='1'  interface=None  automatic_assignment=on  address_offset=hex2dec('00')  intf_name=''  intf_description=''  timing_constraint=None  locs_specified=off  LOCs={'A14'}  io_standard={}  block_type=gatewayout
  data_out : Outport
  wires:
  munge_in/1(dout) -> convert_din1/1, sim_mem/2(data)
  we/1 -> convert_we/1, sim_mem/3(we)
  addr/1 -> calc_add/1(in)
  convert_we/1 -> tut_adc_dac_adc_in_snap_ss_bram_we/1
  tut_adc_dac_adc_in_snap_ss_bram_addr/1 -> Terminator/1
  tut_adc_dac_adc_in_snap_ss_bram_data_in/1 -> Terminator1/1
  tut_adc_dac_adc_in_snap_ss_bram_we/1 -> Terminator2/1
  calc_add/1(out) -> convert_addr/1, sim_mem/1(addr)
  data_in/1 -> munge_in/1(din)
  convert_din1/1 -> tut_adc_dac_adc_in_snap_ss_bram_data_in/1
  convert_addr/1 -> tut_adc_dac_adc_in_snap_ss_bram_addr/1
  tut_adc_dac_adc_in_snap_ss_bram_data_out/1 -> munge_out/1(din)
  sim_mem/1(data_out) -> tut_adc_dac_adc_in_snap_ss_bram_data_out/1
  munge_out/1(dout) -> data_out/1

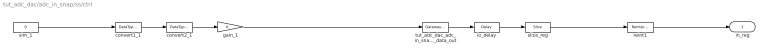
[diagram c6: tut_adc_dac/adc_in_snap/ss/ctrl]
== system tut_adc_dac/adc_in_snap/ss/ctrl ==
  convert1_1 : DataTypeConversion  OutDataTypeStr=fixdt('ufix32_En0')
  convert2_1 : DataTypeConversion  OutDataTypeStr=fixdt('ufix32_En0')  ConvertRealWorld=Stored Integer (SI)
  gain_1 : Gain
  io_delay : xbsIndex_r4/Delay  rst=off  infoeditControl=Selection of Reset will increase slice count due to use of real FFs and instead of SRLs  en=off  latency=0  reg_retiming=on  dbl_ovrd=off  block_type=delay
  reint1 : xbsIndex_r4/Reinterpret  force_arith_type=on  arith_type=Unsigned  force_bin_pt=on  bin_pt=0  block_type=reinterpret
  sim_1 : Constant  Value=0
  slice_reg : xbsIndex_r4/Slice  nbits=32  boolean_output=off  mode=Lower Bit Location + Width  bit1=0  base1=MSB of Input  bit0=0  base0=LSB of Input  dbl_ovrd=off  block_type=slice
  tut_adc_dac_adc_in_snap_ss_ctrl_user_data_out : xbsIndex_r4/Gateway In  gui_display_data_type=Fixed-point  arith_type=Unsigned  n_bits=32  bin_pt=0  preci_type=Single  exp_width=8  frac_width=24  rows=1  columns=1  quantization="Round  (unbiased: +/- Inf)"  overflow=Saturate  period=1  UseAsADC=off  ADCChannel='1'  interface=None  automatic_assignment=on  address_offset=hex2dec('00')  intf_name=''  intf_description=''  default_value=0  timing_constraint=None  locs_specified=off  LOCs={}  io_standard={}  inherit_from_input=off  hdl_port=on  dbl_ovrd=off  block_type=gatewayin
  in_reg : Outport
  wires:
  tut_adc_dac_adc_in_snap_ss_ctrl_user_data_out/1 -> io_delay/1
  sim_1/1 -> convert1_1/1
  convert1_1/1 -> convert2_1/1
  convert2_1/1 -> gain_1/1
  gain_1/1 -> tut_adc_dac_adc_in_snap_ss_ctrl_user_data_out/1
  io_delay/1 -> slice_reg/1
  slice_reg/1 -> reint1/1
  reint1/1 -> in_reg/1

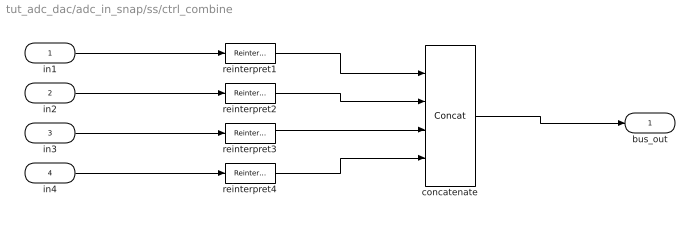
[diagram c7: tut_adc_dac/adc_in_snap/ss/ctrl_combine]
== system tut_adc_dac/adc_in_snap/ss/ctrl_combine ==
  in1 : Inport
  in2 : Inport  Port=2
  in3 : Inport  Port=3
  in4 : Inport  Port=4
  concatenate : xbsIndex_r4/Concat  num_inputs=4  dbl_ovrd=off  block_type=concat
  reinterpret{1..4} (4 alike) : xbsIndex_r4/Reinterpret  force_arith_type=on  arith_type=Unsigned  force_bin_pt=on  bin_pt=0  block_type=reinterpret
  bus_out : Outport
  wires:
  concatenate/1 -> bus_out/1
  in1/1 -> reinterpret1/1
  reinterpret1/1 -> concatenate/1
  in2/1 -> reinterpret2/1
  reinterpret2/1 -> concatenate/2
  in3/1 -> reinterpret3/1
  reinterpret3/1 -> concatenate/3
  in4/1 -> reinterpret4/1
  reinterpret4/1 -> concatenate/4
